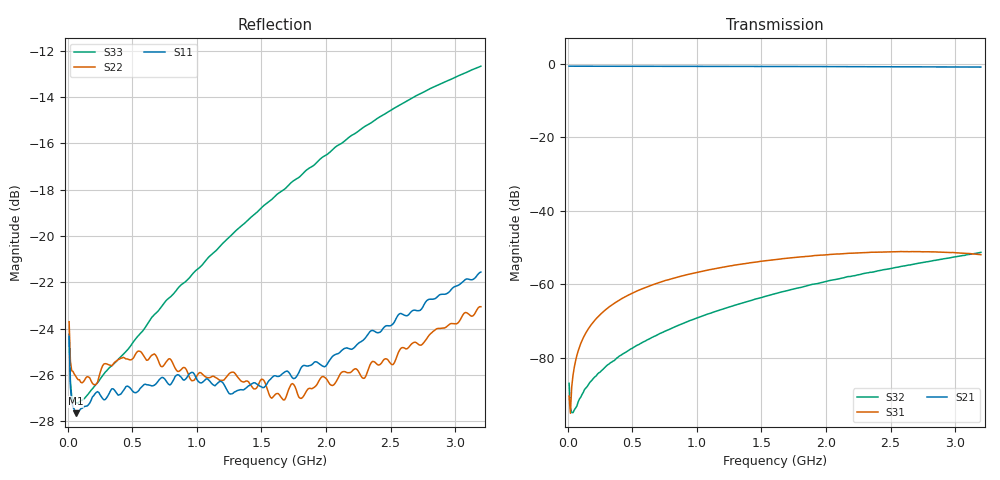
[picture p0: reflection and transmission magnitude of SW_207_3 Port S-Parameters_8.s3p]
! Created _Nov-02-2022_09-58-32
! Type : General
! Retest Level : 0
! Program : FASTESt Rev. 859
! DUT_TempC = 25.0
! Set_V1_Supply_V = 3.0
! V1_Supply_V = 3.0015
! V1_Supply_I = -5e-06
! Set_V2_Supply_V = 0.0
! V2_Supply_V = -0.001
! V2_Supply_I = -3e-06
! RunID = 8
! SN = 4
! Comment = SW-207_SB4_RFc-RF1_room
! Input_Power = 5.0
! Measurement_Comment = None
! Freq	S11db	S11deg	S12db	S12deg	S13db	S13deg	S21db	S21deg	S22db	S22deg	S23db	S23deg	S31db	S31deg	S32db	S32deg	S33db	S33deg
# Hz S dB R 50
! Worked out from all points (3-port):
!   320 points, 10 MHz to 3.2 GHz, reference 50 ohm
!   strongest paths, dB at 10 MHz, 810 MHz, 1.61 GHz, 2.41 GHz, 3.2 GHz:
!     S21: -0.6, -0.6, -0.7, -0.7, -0.8
!     S31: -90.5, -58.5, -53.3, -51.2, -51.9
!     S32: -87.0, -71.9, -62.5, -56.3, -51.3
!   lowest |S11| = -27.7 dB at 60 MHz (marker M1), VSWR 1.09, Z = 54.2 - j1.08 ohm
!   |S11| at or under -10 dB: start of sweep to end of sweep
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1e7  -24.34 -43.2  -0.59 1.3  -90.41 -125.6
     -0.59 1.3  -23.71 -39.7  -87.09 -113.4
     -90.49 -123.0  -86.99 -112.5  -24.26 -38.8
6e7  -27.66 -13.8  -0.60 -5.1  -80.81 80.8
     -0.60 -5.1  -26.05 -12.3  -93.41 -93.0
     -80.90 80.0  -93.71 -93.6  -27.20 -8.7
1.7e8  -27.22 -11.3  -0.61 -15.1  -71.55 73.6
       -0.61 -15.1  -26.13 -10.6  -87.13 -117.8
       -71.56 73.5  -86.78 -117.7  -26.74 -1.4
3.2e8  -26.81 -17.7  -0.62 -28.4  -66.20 62.2
       -0.62 -28.4  -25.57 -18.2  -81.78 -141.3
       -66.17 62.1  -81.70 -141.1  -25.70 -1.2
8.8e8  -26.11 -70.5  -0.64 -77.5  -57.81 18.2
       -0.63 -77.5  -25.76 -68.0  -70.93 149.2
       -57.77 18.2  -70.89 149.4  -22.10 -25.8
1.23e9  -26.62 -114.1  -0.65 -108.1  -55.16 -9.3
        -0.65 -108.1  -26.08 -110.0  -66.48 113.6
        -55.19 -9.4  -66.42 113.8  -20.16 -50.5
1.61e9  -26.04 -163.3  -0.68 -141.3  -53.30 -39.4
        -0.67 -141.4  -26.83 -159.1  -62.59 79.8
        -53.29 -39.5  -62.52 79.9  -18.26 -80.0
2.31e9  -24.37 107.4  -0.74 157.5  -51.39 -94.8
        -0.73 157.5  -26.04 106.9  -57.03 22.5
        -51.37 -94.9  -56.95 22.5  -15.24 -136.5
2.78e9  -22.80 54.5  -0.79 116.4  -51.19 -131.4
        -0.78 116.3  -24.44 51.8  -53.93 -12.7
        -51.15 -131.6  -53.88 -13.0  -13.72 -174.9
3.2e9  -21.56 8.6  -0.84 79.6  -51.97 -162.6
       -0.84 79.5  -23.06 7.8  -51.34 -42.7
       -51.94 -163.0  -51.31 -42.8  -12.67 149.9
